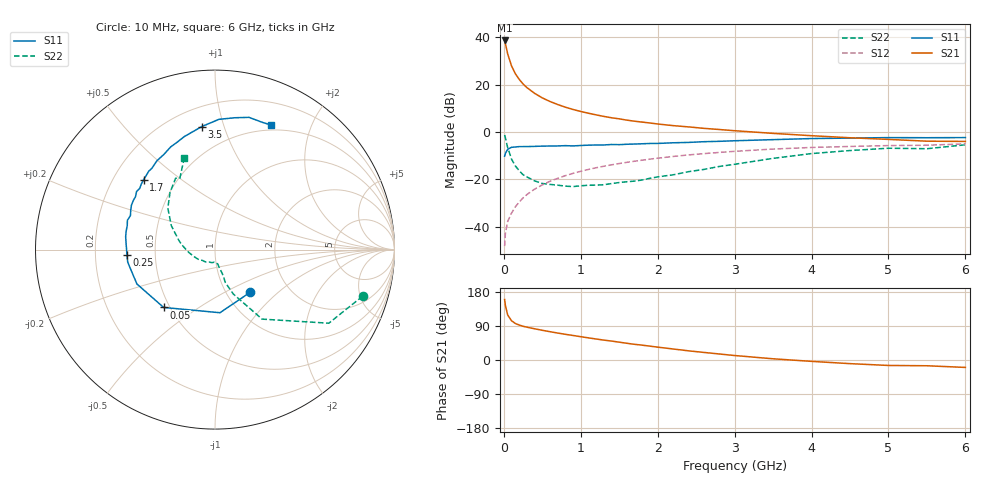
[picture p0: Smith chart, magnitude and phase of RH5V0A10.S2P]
! SIEMENS Small Signal Semiconductors
! BFR106
! Si NPN RF Bipolar Junction Transistor in SOT23
! VCE = 5 V  IC = 100 mA
! Common Emitter S-Parameters:  August  1996
# GHz  S  MA  R  50
!  f  S11  S21  S12  S22
! GHz  MAG  ANG  MAG  ANG  MAG  ANG  MAG  ANG
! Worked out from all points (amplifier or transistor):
!   36 points, 10 MHz to 6 GHz, reference 50 ohm
!   highest |S21| = 38.6 dB at 10 MHz (marker M1)
!   |S21| within 3 dB of that: start of sweep to 31.77 MHz
!   unconditionally stable (mu >= 1): 167.3 MHz to 2.465 GHz; 5.439 GHz to 5.668 GHz
!   at 250 MHz: K = 1.06, MAG = 22.5 dB, |S12| = -27.8 dB
!   at 1.4 GHz: K = 1.07, MAG = 8.3 dB, |S12| = -13.9 dB
!   at 6 GHz: K = 0.99, MSG = 0.5 dB, |S12| = -5.0 dB
!   S11 on the Smith chart (normalised r, x): 10 MHz: 1.28, -0.68; 50 MHz: 0.46, -0.37; 250 MHz: 0.34, -0.03; 1.7 GHz: 0.33, +0.37; 3.5 GHz: 0.32, +0.84; 6 GHz: 0.44, +1.46
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0.01  0.3081 -50.8  85.19 159.7  0.0039 78.2  0.8625 -17.5
0.02  0.3528 -85.5  73.63 144.1  0.0072 71.2  0.7551 -32.9
0.05  0.431 -131.6  44.26 118.8  0.013 60.7  0.4677 -55.9
0.1  0.4753 -156.2  24.75 103.6  0.0194 65.3  0.2677 -67.6
0.15  0.4824 -166.8  16.9 96.3  0.0265 67.9  0.1919 -72.6
0.2  0.4912 -171.9  12.85 92.3  0.0332 71.1  0.1521 -72.5
0.25  0.4915 -176.3  10.29 89.0  0.0408 71.9  0.1252 -74.2
0.3  0.4921 -178.9  8.624 86.6  0.0478 73.8  0.1127 -75.7
0.4  0.4965 176.0  6.528 82.4  0.0623 74.1  0.093 -77.6
0.5  0.5029 171.8  5.233 78.4  0.0763 74.0  0.0819 -79.0
0.6  0.5055 168.4  4.396 74.7  0.0913 73.1  0.0783 -82.2
0.7  0.507 164.6  3.793 71.1  0.1052 72.0  0.0755 -87.0
0.8  0.5147 161.5  3.332 67.8  0.1198 70.6  0.072 -91.4
1.1  0.5271 152.1  2.483 58.4  0.162 66.9  0.0752 -106.1
1.3  0.5318 146.4  2.128 52.5  0.1893 64.0  0.0772 -116.1
1.7  0.5567 135.5  1.686 41.4  0.2417 58.1  0.092 -138.8
2.2  0.5915 123.1  1.361 29.1  0.3042 50.4  0.1248 -162.8
2.8  0.6348 109.3  1.127 15.9  0.3701 41.0  0.1872 171.6
3.5  0.6891 96.2  0.934 3.2  0.4364 30.4  0.2776 151.3
4.5  0.7427 81.5  0.755 -9.6  0.4949 15.6  0.4056 128.1
5.5  0.7565 69.5  0.639 -15.2  0.525 6.0  0.4432 116.2
6  0.7612 65.7  0.632 -19.6  0.562 -1.0  0.5364 108.7
